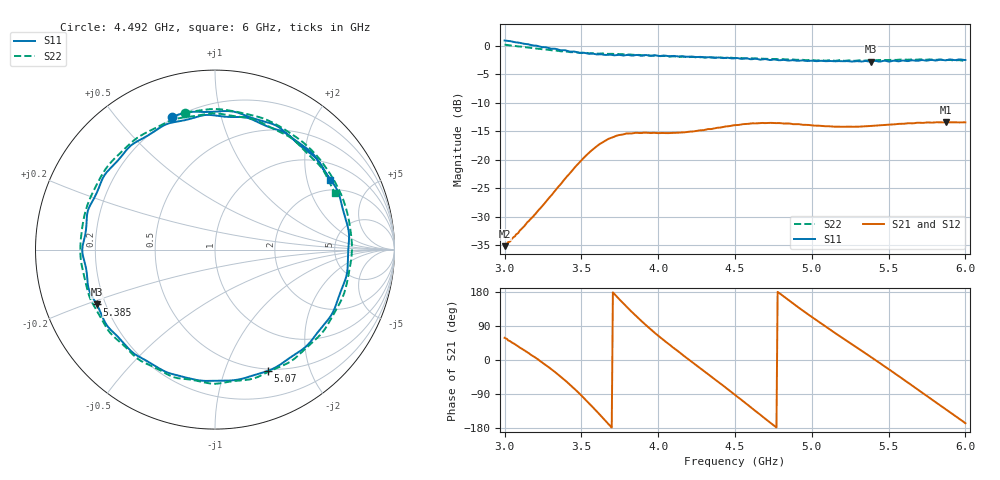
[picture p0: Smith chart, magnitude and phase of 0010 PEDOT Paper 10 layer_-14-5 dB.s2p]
!  04/11/2025  20:13:34
! Ref Plane: 0.000 mm
# MHZ S MA R  50
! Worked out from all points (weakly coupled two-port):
!   401 points, 3 GHz to 6 GHz, reference 50 ohm
!   highest |S21| = -13.42 dB at 5.872 GHz (marker M1); lowest = -35.2 dB at 3 GHz (marker M2)
!   lowest |S11| = -2.8 dB at 5.385 GHz (marker M3), VSWR 6.30, Z = 8.32 - j10.8 ohm
!   |S11| at or under -10 dB: nowhere
!   |S22| runs from -2.7 to 0.2 dB; largest |S21 - S12| = 0.0045
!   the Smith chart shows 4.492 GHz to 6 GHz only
!   S11 on the Smith chart (normalised r, x): 4.492 GHz: 0.19, +0.71; 5.07 GHz: 0.48, -1.42; 5.385 GHz: 0.17, -0.22; 6 GHz: 1.57, +2.79
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3000  1.114 -112.5  0.0174 58.5  0.01748 59.9  1.024 -117.0
3270  0.9708 -179.9  0.04311 -13.7  0.04297 -12.7  0.9269 175.7
3390  0.9149 142.7  0.06721 -52.3  0.06746 -51.9  0.8943 137.7
3502.5  0.8696 100.6  0.0996 -94.8  0.09973 -94.4  0.8677 95.2
3607.5  0.8398 56.5  0.1336 -138.7  0.1338 -138.5  0.8525 51.4
3735  0.831 0.1  0.1633 165.4  0.1636 166.2  0.8452 -4.1
3870  0.8282 -54.5  0.1718 110.4  0.1731 111.3  0.8325 -58.3
4005  0.8142 -102.0  0.1711 62.8  0.1709 63.5  0.8135 -105.0
4237.5  0.7985 -174.3  0.1778 -10.7  0.1778 -9.7  0.795 -177.4
4357.5  0.7866 149.7  0.1872 -47.4  0.1878 -46.3  0.7897 145.5
4492.5  0.776 107.8  0.2005 -89.8  0.2021 -89.0  0.781 102.3
4500  0.7792 105.4  0.201 -92.3  0.2023 -91.6  0.78 99.6
4612.5  0.7631 70.5  0.2086 -127.9  0.209 -127.6  0.7757 63.0
4755  0.7575 26.3  0.2092 -173.5  0.2096 -172.7  0.765 16.4
5002.5  0.7405 -47.2  0.1998 112.8  0.1995 113.4  0.7504 -58.0
5070  0.7372 -66.5  0.1973 93.9  0.197 94.3  0.7458 -77.0
5227.5  0.7343 -111.0  0.195 50.6  0.1952 51.0  0.7411 -120.5
5385  0.7259 -155.1  0.1978 7.8  0.1983 8.6  0.7456 -162.1
5505  0.727 171.4  0.2031 -25.3  0.204 -24.3  0.752 164.8
5700  0.7433 115.4  0.2111 -80.9  0.2122 -79.9  0.7596 110.0
5872.5  0.7459 66.7  0.2132 -130.5  0.2144 -129.6  0.7485 61.2
6000  0.7508 31.1  0.2124 -166.9  0.2132 -166.3  0.7382 25.1
